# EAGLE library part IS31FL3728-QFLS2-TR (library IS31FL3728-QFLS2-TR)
LED Lighting Drivers Audio Mod Matrix LED Driver Source: Datasheet
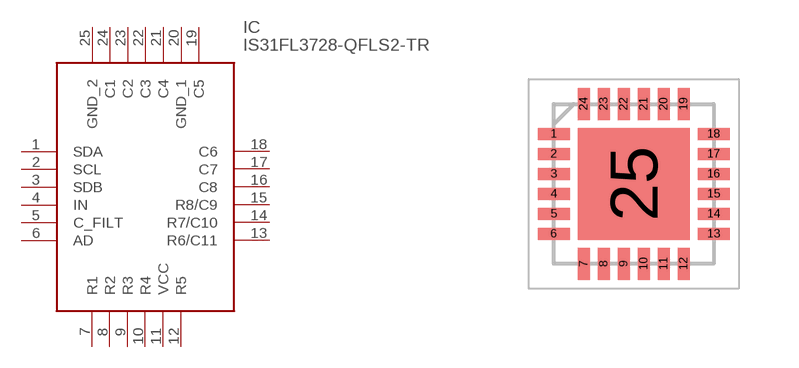
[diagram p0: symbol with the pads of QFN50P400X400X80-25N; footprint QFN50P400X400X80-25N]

Designator prefix IC

## IS31FL3728-QFLS2-TR (Arrow_Part_Number: IS31FL3728-QFLS2-TR; Arrow_Price-Stock: https://www.arrow.com/en/products/is31fl3728-qfls2-tr/integrated-silicon-solution-inc; Description: LED Lighting Drivers Audio Mod Matrix LED Driver; Height: 0.8mm; Manufacturer_Name: Integrated Silicon Solution Inc.; Manufacturer_Part_Number: IS31FL3728-QFLS2-TR; Mouser_Part_Number: 870-IS31FL3728QFLS2R; Mouser_Price-Stock: https://www.mouser.com/Search/Refine.aspx?Keyword=870-IS31FL3728QFLS2R)  [QFN50P400X400X80-25N]
1  SDA
2  SCL
3  SDB
4  IN
5  C_FILT
6  AD
7  R1
8  R2
9  R3
10  R4
11  VCC
12  R5
13  R6/C11
14  R7/C10
15  R8/C9
16  C8
17  C7
18  C6
19  C5
20  GND_1
21  C4
22  C3
23  C2
24  C1
25  GND_2

## Footprint QFN50P400X400X80-25N (pad centres in mm)
IS31FL3728-QFLS2-TR
smd 0.8 x 0.3: 1 -2,1.25; 2 -2,0.75; 3 -2,0.25; 4 -2,-0.25; 5 -2,-0.75; 6 -2,-1.25; 13 2,-1.25; 14 2,-0.75; 15 2,-0.25; 16 2,0.25; 17 2,0.75; 18 2,1.25
smd 0.3 x 0.8: 7 -1.25,-2; 8 -0.75,-2; 9 -0.25,-2; 10 0.25,-2; 11 0.75,-2; 12 1.25,-2; 19 1.25,2; 20 0.75,2; 21 0.25,2; 22 -0.25,2; 23 -0.75,2; 24 -1.25,2
smd 2.8 x 2.8: 25 0,0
